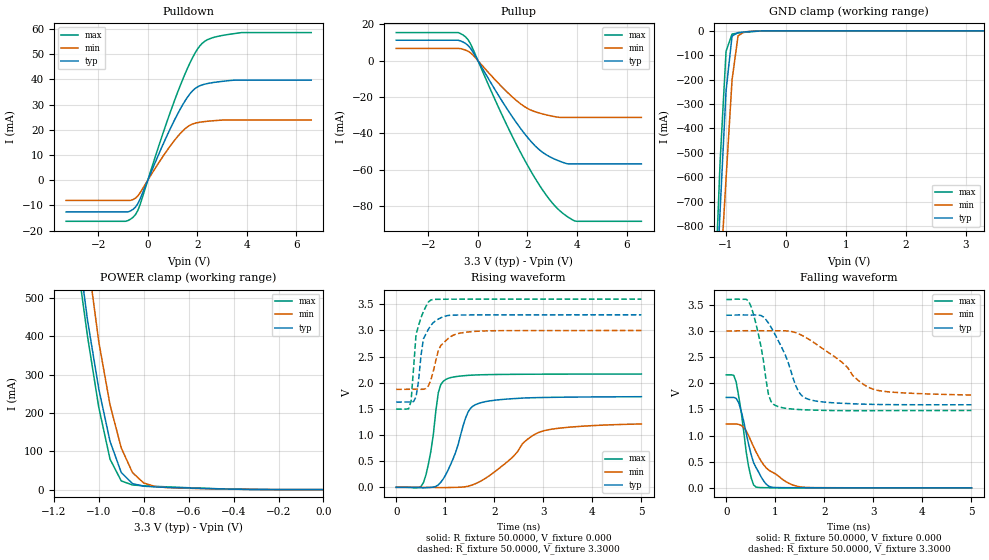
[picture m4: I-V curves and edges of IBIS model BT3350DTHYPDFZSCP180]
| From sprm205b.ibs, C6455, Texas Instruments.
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|   Model BT3350DTHYPDFZSCP180
[Model]   BT3350DTHYPDFZSCP180
Model_type   I/O
Polarity   Non-Inverting
Enable   Active-Low
Vinl =   0.8000V
Vinh =   2.0000V
Vmeas =   1.5000V
Cref =  10.0000pF
Rref =  50.0000
Vref =   1.5000V
C_comp   1.3625pF   1.3089pF   1.4308pF
[Temperature Range]   25.0000   0.1250k   -40.0000
[Pullup Reference]   3.3000V   3.0000V   3.6000V
[Pulldown Reference]   0.000V   0.000V   0.000V
[POWER Clamp Reference]   3.3000V   3.0000V   3.6000V
[GND Clamp Reference]   0.000V   0.000V   0.000V
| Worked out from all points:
|   slope of the pulldown table from 0 to 0.495 V, typ, clamps not added: 42.9 ohm
|   slope of the pullup table from 0 to 0.495 V, typ, clamps not added: 42.8 ohm
|   GND clamp passes 1 mA (typ) near -0.47 V on its own axis
|   POWER clamp passes 1 mA (typ) near -0.38 V on its own axis
|   rising waveform, R_fixture 50.0000, V_fixture 0.000: 20-80 % time 375ps typ, 822ps min, 194ps max; typ from 0 V to 1.73 V
|   rising waveform, R_fixture 50.0000, V_fixture 3.3000: 20-80 % time 181ps typ, 257ps min, 158ps max; typ from 1.63 V to 3.3 V
|   falling waveform, R_fixture 50.0000, V_fixture 0.000: 20-80 % time 307ps typ, 570ps min, 194ps max; typ from 1.73 V to 0 V
|   falling waveform, R_fixture 50.0000, V_fixture 3.3000: 20-80 % time 449ps typ, 916ps min, 245ps max; typ from 3.3 V to 1.59 V
[Pulldown]
| voltage   I(typ)   I(min)   I(max)
-3.3V     -12.59mA   -8.027mA   -16.31mA
-800mV    -12.59mA   NA         -16.01mA
-500mV    -10.71mA   -7.129mA   -13.69mA
-300mV    -7.174mA   -4.816mA   -9.34mA
600mV     13.87mA    9.263mA    18.23mA
1.3V      28.03mA    18.4mA     37.29mA
1.6V      32.9mA     21.17mA    44.34mA
1.9V      36.3mA     22.58mA    50.31mA
2.3V      38.1mA     23.27mA    55.11mA
2.7V      38.83mA    23.63mA    56.76mA
3.5V      39.68mA    NA         58.17mA
6.6V      39.68mA    23.89mA    58.57mA
[Pullup]
| voltage   I(typ)   I(min)   I(max)
-3.3V     11.22mA    6.705mA    15.43mA
-800mV    11.22mA    6.705mA    15.43mA
-500mV    9.448mA    5.765mA    13.06mA
-300mV    6.8mA      4.288mA    9.245mA
1V        -22.82mA   -14.89mA   -30.69mA
2V        -42.2mA    -26.3mA    -57.53mA
2.4V      -48.09mA   -28.53mA   -66.74mA
2.8V      -52.15mA   -29.97mA   -74.81mA
3.2V      -54.81mA   -31.07mA   -81.26mA
3.5V      -56.34mA   NA         -84.78mA
3.7V      -56.87mA   NA         -86.64mA
6.6V      -56.87mA   -31.26mA   -88.43mA
[GND_clamp]
| voltage   I(typ)   I(min)   I(max)
-3.3V     -15.87A    -14.34A    -17.08A
-1.2V     -1.264A    -1.455A    -1.162A
-1.1V     -739.7mA   -1.022A    -540mA
-1V       -245.4mA   -606.2mA   -83.6mA
-900mV    -21.55mA   -201.1mA   -13.2mA
-800mV    -7.093mA   -20.73mA   -8.982mA
-700mV    -4.696mA   -4.545mA   -6.387mA
-300mV    -39.42uA   -55.51uA   -61.72uA
3.3V      64.17uA    87.18uA    296.3nA
[POWER_clamp]
| voltage   I(typ)   I(min)   I(max)
-3.3V     13.83A     12.48A     14.95A
-1.1V     665.8mA    853.9mA    613.8mA
-1.05V    441.7mA    607.3mA    399.5mA
-1V       262.6mA    385.7mA    214.6mA
-950mV    126.1mA    221.3mA    79.57mA
-900mV    44.61mA    108.8mA    22.66mA
-850mV    15.61mA    44.43mA    12.1mA
-800mV    8.911mA    17.17mA    9.881mA
-750mV    7.015mA    8.23mA     8.52mA
-650mV    4.984mA    4.132mA    6.055mA
-350mV    700.6uA    798uA      623.7uA
0V        336.1nA    1.596uA    433.6nA
[Ramp]
| variable   typ   min   max
dV/dt_r   1.0399/0.3715n   0.7269/0.8632n   1.3004/0.1917n
dV/dt_f   1.0270/0.4450n   0.7349/0.9570n   1.2725/0.2431n
R_load = 50.0000
[Rising Waveform]
R_fixture = 50.0000
V_fixture = 0.000
V_fixture_min = 0.000
V_fixture_max = 0.000
| time   V(typ)   V(min)   V(max)
0s        42.92uV    34.49uV    82.66uV
555.6ps   -9.527mV   -346.9uV   90.76mV
707.1ps   -1.496mV   -1.498mV   691.1mV
858.6ps   47.56mV    -5.678mV   1.81V
1.01ns    241.3mV    -5.196mV   2.063V
1.212ns   669.9mV    -650uV     2.117V
1.465ns   1.438V     20.52mV    2.141V
1.667ns   1.6V       91.39mV    2.151V
2.929ns   1.717V     1.058V     2.164V
5ns       1.733V     1.212V     2.167V
[Rising Waveform]
R_fixture = 50.0000
V_fixture = 3.3000
V_fixture_min = 3.0000
V_fixture_max = 3.6000
| time   V(typ)   V(min)   V(max)
0s        1.631V     1.874V     1.496V
252.5ps   1.632V     1.875V     1.503V
303ps     1.631V     1.876V     1.646V
404ps     1.731V     1.875V     2.921V
454.5ps   2.028V     1.875V     3.09V
555.6ps   2.84V      1.876V     3.362V
707.1ps   3.1V       2.052V     3.585V
909.1ps   3.243V     2.711V     3.597V
1.263ns   3.296V     2.941V     3.599V
5ns       3.3V       2.999V     3.6V
[Falling Waveform]
R_fixture = 50.0000
V_fixture = 0.000
V_fixture_min = 0.000
V_fixture_max = 0.000
| time   V(typ)   V(min)   V(max)
0s        1.728V     1.22V      2.16V
151.5ps   1.729V     1.22V      2.151V
202ps     1.709V     1.22V      2.018V
303ps     1.466V     1.194V     1.454V
454.5ps   831.5mV    997.6mV    405.5mV
555.6ps   483mV      784.4mV    57.54mV
606.1ps   388mV      687mV      13.79mV
858.6ps   35.81mV    344mV      2.559mV
1.465ns   2.187mV    26.04mV    577.7uV
5ns       128.3uV    684.5uV    2.724uV
[Falling Waveform]
R_fixture = 50.0000
V_fixture = 3.3000
V_fixture_min = 3.0000
V_fixture_max = 3.6000
| time   V(typ)   V(min)   V(max)
0s        3.3V       3V         3.6V
454.5ps   3.303V     3.003V     3.569V
656.6ps   3.303V     3.003V     2.926V
858.6ps   3.151V     3.002V     1.79V
1.01ns    2.902V     3.002V     1.571V
1.212ns   2.517V     3.001V     1.52V
1.465ns   1.856V     2.949V     1.498V
1.667ns   1.695V     2.849V     1.489V
2.98ns    1.596V     1.891V     1.476V
5ns       1.588V     1.775V     1.479V
